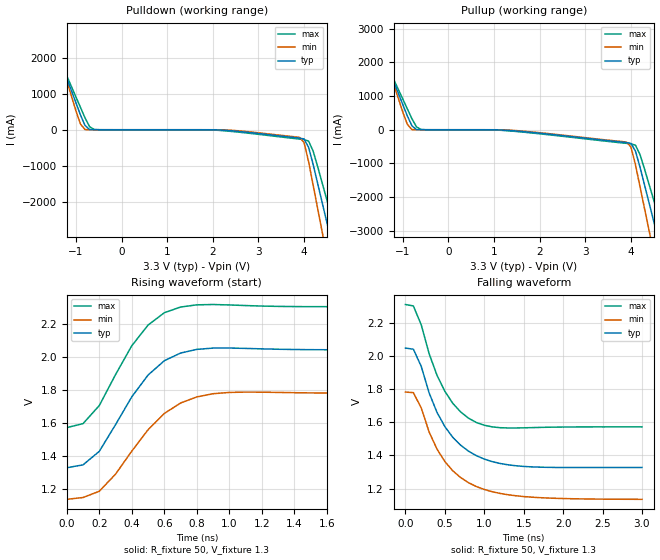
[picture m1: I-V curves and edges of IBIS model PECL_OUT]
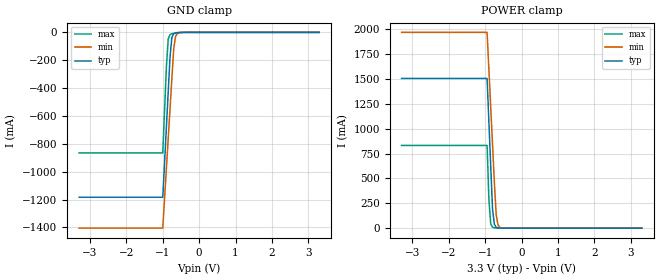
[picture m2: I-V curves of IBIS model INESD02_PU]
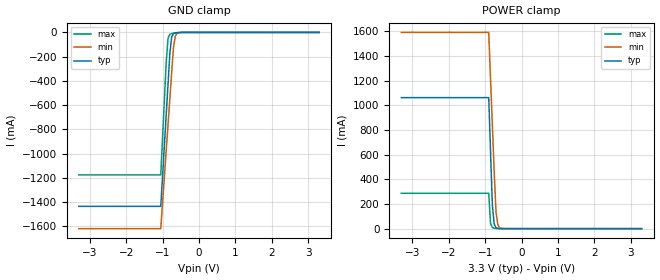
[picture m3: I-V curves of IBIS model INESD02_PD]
|   This file is an IBIS representation of the   |
|   Integrated Device Technology, Inc.   |
|   ICS843204I   |
|   3.3V FemtoClock Crystal-to-3.3V LVPECL Synthesizer   |
[IBIS Ver]   3.2
[File name]   843204i_3v3.ibs
[File Rev]   1.0
[Date]   July 28 2008 | Last modified
|   July 28 2008 | Generated
[Source] Originated at Integrated Device Technology, Inc.
[Disclaimer]
IDT hereby grants the user of this IBIS model a non-exclusive,
nontransferable license to use this IBIS model under the following terms.
Before using this IBIS model, the user should read this license.
If the user does not accept these terms,  the IBIS model should be
returned to IDT within 30 days.
   The user is granted this license only to use the IBIS model and
is not granted rights to sell, load, rent, lease or license the IBIS
model in whole or in part, or in modified form to anyone other than
user. User may modify the IBIS model to suit its specific
applications but rights to derivative works and such modifications
shall belong to ICS.
   This IBIS model is provided on an "AS IS" basis and IDT makes
absolutely no warranty with respect to the information contained
herein. IDT DISCLAIMS AND CUSTOMER WAIVES ALL WARRANTIES, EXPRESS
OR IMPLIED, INCLUDING WARRANTIES OF MERCHANTABILITY OR FITNESS FOR
A PARTICULAR PURPOSE. The entire risk as to quality and performance
is with the Customer. ACCORDINGLY, IN NO EVENT SHALL THE COMPANY BE
LIABLE FOR ANY DAMAGES, WHETHER IN CONTRACT OR TORT,INCLUDING ANY
LOST PROFITS OR OTHER INCIDENTAL, CONSEQUENTIAL, EXEMPLARY, OR
PUNITIVE DAMAGES ARISING OUT OF THE USE OR APPLICATION OF THE IBIS
model provided in this package. Further, IDT reserves the right to
make changes without notice to any product herein to improve
reliability, function, or design. IDT does not convey any license
under patent rights or any other intellectual property rights,
including those of third parties.
   IDT is not obligated to provide maintenance or support
for the licensed IBIS model.
[Copyright]   Copyright 2008 by Integrated Device Technology, Inc.
[Component]   ICS843204AGI
[Manufacturer] Integrated Device Technology, Inc.
[Package]
|TSSOP 48 Pin
|   typ   min   max
R_pkg   88.2m   76.6m   99.8m
L_pkg   3.369nH   2.250nH   4.488nH
C_pkg   0.548pF   0.377pF   0.718pF
[Pin]   signal_name   model_name
1   nQA1   PECL_OUT
2   QA1   PECL_OUT
3   nQA0   PECL_OUT
4   QA0   PECL_OUT
|5   nc
6   VCCO_A   POWER
7   SELA1   INESD02_PD
8   SELA0   INESD02_PD
9   nPLL_BYPASS_A   INESD02_PU
|10   nc
|11   nc
|12   nc
|13   nc
|14   XTAL_IN1
|15   XTAL_OUT1
16   CLK1   INPUT_PD_CLK
17   IN_SEL_B   INESD02_PU
18   nPLL_BYPASS_B   INESD02_PU
19   VCCO_B   POWER
|20   nc
21   QB0   PECL_OUT
22   nQB0   PECL_OUT
23   QB1   PECL_OUT
24   nQB1   PECL_OUT
|25   nc
|26   nc
|27   nc
|28   nc
|29   nc
30   VCCA_B   POWER
31   SELB1   INESD02_PD
32   VCC   POWER
33   OEB1   INESD02_PU
34   OEB0   INESD02_PU
35   VEE   GND
36   SELB0   INESD02_PD
|37   nc
|38   nc
39   VCCA_A   POWER
40   VCC   POWER
41   OEA1   INESD02_PU
42   OEA0   INESD02_PU
43   VEE   GND
|44   nc
|45   XTAL_OUT0
|46   XTAL_IN0
47   CLK0   INPUT_PD_CLK
48   IN_SEL_A   INESD02_PU
[Diff Pin]  inv_pin  vdiff tdelay_typ tdelay_min  tdelay_max
2   1   NA   0   0   0
4   3   NA   0   0   0
22   21   NA   0   0   0
24   23   NA   0   0   0
| Models and submodels in the file (4): PECL_OUT (Output_ECL), INESD02_PU (Input), INESD02_PD (Input), INPUT_PD_CLK (Input)
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[Model]   PECL_OUT
Model_type  Output_ECL
Polarity   Non-Inverting
Vmeas = 1.7
Rref = 50
Cref = 0
Vref = 1.3
|Variable  typ   min   max
C_comp   2p   1.5p   2.5p
[Voltage Range]   3.3   3.135   3.465
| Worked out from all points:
|   rising waveform, R_fixture 50, V_fixture 1.3: 20-80 % time 285ps typ, 317ps min, 265ps max; typ from 1.33 V to 2.05 V
|   falling waveform, R_fixture 50, V_fixture 1.3: 20-80 % time 459ps typ, 483ps min, 378ps max; typ from 2.05 V to 1.33 V
|  Voltage   I(typ)   I(min)   I(max)
[Pullup]
-3.3V     8.64A      10.19A     7.67A
-1.8V     3.488A     3.876A     3.257A
-1.6V     2.802A     3.037A     2.67A
-1V       750.7mA    525.2mA    911.8mA
-800mV    117.7mA    4.129mA    328.1mA
-600mV    578.7uA    8.433uA    7.697mA
3.9V      -381mA     -366.1mA   -404mA
4.1V      -638.2mA   -1.044A    -460.5mA
4.4V      -2.187A    -3.01A     -1.635A
4.6V      -3.257A    -4.321A    -2.553A
4.7V      -3.793A    -4.976A    -3.011A
6.6V      -13.98A    -17.46A    -11.73A
[Pulldown]
-3.3V     8.64A      10.19A     7.67A
-1.6V     2.802A     3.037A     2.67A
-900mV    410.1mA    159.1mA    619.7mA
-800mV    117.7mA    4.129mA    328.1mA
-600mV    578.7uA    8.433uA    7.697mA
3.9V      -231.9mA   -211.3mA   -258.3mA
4V        -255.6mA   -354.4mA   -273.3mA
4.1V      -489mA     -888.6mA   -314.9mA
4.4V      -2.037A    -2.854A    -1.49A
4.6V      -3.108A    -4.165A    -2.407A
4.7V      -3.643A    -4.82A     -2.866A
6.6V      -13.87A    -17.38A    -11.61A
[Ramp]
|   typ   min   max
dV/dt_r   0.45V/0.37ns   0.45V/0.405ns   0.45V/0.27ns
dV/dt_f   0.45V/0.37ns   0.45V/0.405ns   0.45V/0.27ns
R_load =   50.0000
[Rising Waveform]
R_fixture = 50
V_fixture = 1.3   | VCC_typ - 2V
V_fixture_max = 1.465   | VCC_max - 2V
V_fixture_min = 1.135   | VCC_min - 2V
C_fixture = 0.0p
| Time   typ   min   max
0s        1.328V     1.136V     1.572V
100ps     1.345V     1.147V     1.597V
200ps     1.428V     1.185V     1.706V
300ps     1.59V      1.289V     1.895V
400ps     1.76V      1.429V     2.071V
500ps     1.892V     1.559V     2.196V
600ps     1.979V     1.658V     2.272V
700ps     2.026V     1.722V     2.306V
1ns       2.057V     1.786V     2.319V
3ns       2.046V     1.782V     2.309V
[Falling Waveform]
R_fixture = 50
V_fixture = 1.3   | VCC_typ - 2V
V_fixture_max = 1.465   | VCC_max - 2V
V_fixture_min = 1.135   | VCC_min - 2V
C_fixture = 0.0p
| Time   typ   min   max
0s        2.046V     1.782V     2.309V
100ps     2.04V      1.778V     2.3V
200ps     1.936V     1.686V     2.187V
300ps     1.776V     1.542V     2.013V
400ps     1.659V     1.438V     1.883V
500ps     1.574V     1.363V     1.786V
700ps     1.462V     1.267V     1.662V
900ps     1.399V     1.213V     1.598V
1.5ns     1.334V     1.153V     1.567V
3ns       1.328V     1.136V     1.572V
[Model]   INESD02_PU
Model_type   Input
Polarity   Non-Inverting
Vinl = 0.80V
Vinh = 2.0V
|   typ   min   max
C_comp   2pF   1.5pF   2.5pF
|   typ   min   max
[Voltage range]  3.3V   3.15V   3.45V
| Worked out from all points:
|   GND clamp passes 1 mA (typ) near -0.56 V on its own axis
|   POWER clamp passes 1 mA (typ) near -0.61 V on its own axis
[GND_clamp]
|Voltage   I(typ)   I(min)   I(max)
-3.3V     -1.184A    -1.405A    -865.6mA
-1V       -1.184A    -1.405A    -865.6mA
-900mV    -678.5mA   -975.1mA   -244.1mA
-850mV    -426.2mA   -760.2mA   -46.92mA
-800mV    -174mA     -545.4mA   -16.17mA
-750mV    -37.03mA   -330.8mA   -9.981mA
-700mV    -9.767mA   -120.3mA   -7.122mA
-650mV    -3.616mA   -29.78mA   -4.922mA
-600mV    -1.7mA     -7.594mA   -3.115mA
-400mV    -123.9uA   -126uA     -173.9uA
3.3V      1.866nA    3.949uA    0A
[POWER_clamp]
|Voltage   I(typ)   I(min)   I(max)
-3.3V     1.506A     1.97A      832.1mA
-950mV    1.506A     1.97A      832.1mA
-900mV    1.063A     1.592A     287.2mA
-850mV    620.4mA    1.215A     41.77mA
-800mV    191.5mA    837.4mA    8.692mA
-750mV    37.69mA    460.1mA    3.262mA
-700mV    8.032mA    133.8mA    1.662mA
-650mV    2.005mA    32.58mA    840.1uA
-600mV    607uA      8.009mA    378.6uA
-450mV    33.11uA    139.8uA    23.88uA
3.3V      -71.13uA   -77.46uA   -62.11uA
[Model]   INESD02_PD
Model_type   Input
Polarity   Non-Inverting
Vinl = 0.80V
Vinh = 2.0V
|   typ   min   max
C_comp   2pF   1.5pF   2.5pF
|   typ   min   max
[Voltage range]  3.3V   3.15V   3.45V
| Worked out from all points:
|   GND clamp passes 1 mA (typ) near -0.56 V on its own axis
|   POWER clamp passes 1 mA (typ) near -0.61 V on its own axis
[GND_clamp]
|Voltage   I(typ)   I(min)   I(max)
-3.3V     -1.436A    -1.62A     -1.176A
-1.05V    -1.436A    -1.62A     -1.176A
-900mV    -678.5mA   -975.1mA   -244mA
-850mV    -426.1mA   -760.1mA   -46.85mA
-800mV    -173.9mA   -545.4mA   -16.11mA
-750mV    -36.96mA   -330.7mA   -9.916mA
-700mV    -9.696mA   -120.2mA   -7.056mA
-650mV    -3.545mA   -29.7mA    -4.857mA
-600mV    -1.629mA   -7.52mA    -3.049mA
-400mV    -52.81uA   -52.52uA   -108.7uA
3.3V      71.13uA    77.43uA    62.11uA
[POWER_clamp]
|Voltage   I(typ)   I(min)   I(max)
-3.3V     1.063A     1.593A     287.3mA
-900mV    1.063A     1.593A     287.3mA
-850mV    620.5mA    1.215A     41.84mA
-800mV    191.6mA    837.5mA    8.757mA
-750mV    37.76mA    460.2mA    3.328mA
-700mV    8.104mA    133.8mA    1.728mA
-650mV    2.076mA    32.66mA    905.3uA
-600mV    678.1uA    8.083mA    443.8uA
-450mV    104.2uA    213.3uA    89.09uA
3.3V      -3.041nA   -3.986uA   0A
